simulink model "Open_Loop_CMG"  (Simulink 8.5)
settings: Solver=ode45  StartTime=0.0  StopTime=10.0  RelTol=1e-3
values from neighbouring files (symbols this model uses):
  Ave = [    [vehicle_flex34.m]    (also in vehicle_rigid.m)
  Bve = [    [vehicle_flex34.m]    (also in vehicle_rigid.m)
  Cve = [    [vehicle_flex34.m]    (also in vehicle_rigid.m)
  Dve = [    [vehicle_flex34.m]    (also in vehicle_rigid.m)
  J = [0.119416e9, -0.476e7,   -0.1216e7;     -0.476e7,     0.40408e8, -0.30121e6;     -0.1216e7,   -0.30121e6,  0.110166e9]    [start.m]    (also in start1.m; start2.m; start3.m)
  omg = 20*wo    (= 0.022)    [start.m]    (also in start1.m; start2.m; start3.m)
  zeb = 0.95    [start.m]    (also in start1.m; start2.m; start3.m)

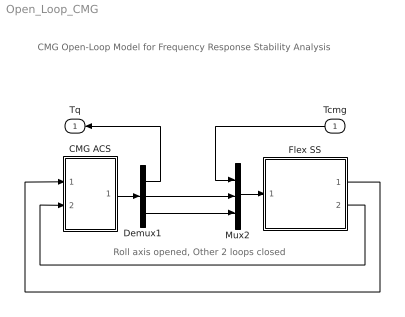
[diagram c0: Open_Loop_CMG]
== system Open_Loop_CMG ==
  note: CMG Open-Loop Model for Frequency Response Stability Analysis
  note: Roll axis opened, Other 2 loops closed
  Tcmg : Inport
  CMG ACS : Subsystem
  Demux1 : Demux  Outputs=3
  Flex SS : Subsystem
  Mux2 : Mux  Inputs=3
  Tq : Outport
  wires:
  Flex SS/2(att) -> CMG ACS/2(ater)
  Flex SS/1(wb) -> CMG ACS/1(wb)
  Mux2/1 -> Flex SS/1(Tcmg)
  CMG ACS/1(Tq) -> Demux1/1
  Demux1/2 -> Mux2/2
  Demux1/3 -> Mux2/3
  Demux1/1 -> Tq/1
  Tcmg/1 -> Mux2/1

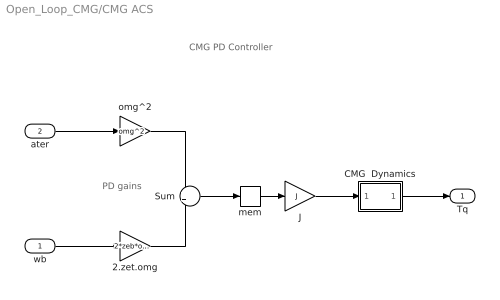
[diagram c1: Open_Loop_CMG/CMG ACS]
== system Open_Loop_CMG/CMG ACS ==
  note: CMG PD Controller
  note: PD gains
  wb : Inport
  ater : Inport  Port=2  PortDimensions=3
  2.zet.omg : Gain  Gain=2*zeb*omg
  CMG  Dynamics : Subsystem
  J : Gain  Gain=J  Multiplication=Matrix(K*u)
  Sum : Sum
  mem : Memory
  omg^2 : Gain  Gain=omg^2
  Tq : Outport
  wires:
  wb/1 -> 2.zet.omg/1
  Sum/1 -> mem/1
  2.zet.omg/1 -> Sum/2
  ater/1 -> omg^2/1
  omg^2/1 -> Sum/1
  J/1 -> CMG  Dynamics/1(I)
  mem/1 -> J/1
  CMG  Dynamics/1(O) -> Tq/1

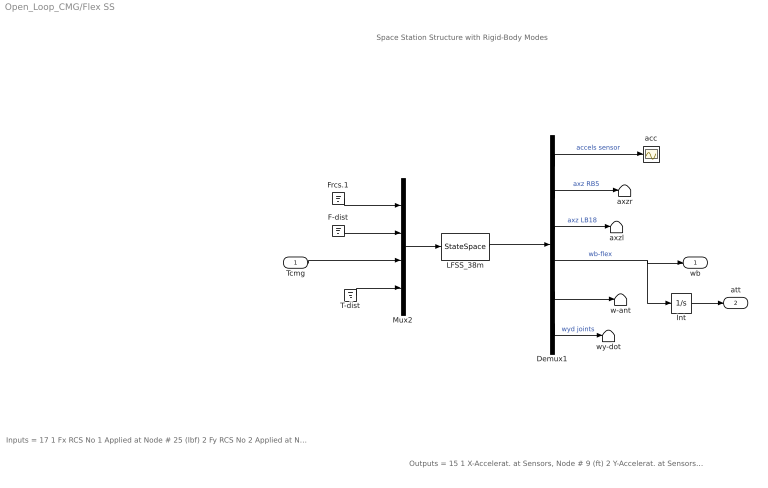
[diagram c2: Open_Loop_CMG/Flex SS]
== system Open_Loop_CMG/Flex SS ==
  note: Space Station Structure with Rigid-Body Modes
  note: Inputs = 17 1 Fx RCS No 1 Applied at Node # 25 (lbf) 2 Fy RCS No 2 Applied at Node # 25 (lbf) 3 Fx RCS No 3 Applied at Node # 26 (lbf) 4 Fy RCS No 4 Applied at Node # 26 (lbf) 5 Fx RCS No 5 Applied at Node # 27 (lbf) 6 Fy RCS No 6 Applied at Node # 27 (lbf) 7 Fx RCS No 7 Applied at Node # 28 (lbf) 8 Fy RCS No 8 Applied at Node # 28 (lbf) 9 Fx Disturb. No 9 at Node # 21 (lbf) 10 Fy Disturb. No 10 at Node # 21 (lbf) 11 Fz Disturb. No 11 at Node # 21 (lbf) 12 Torq-x No 1 CMG Applied at Node # 10 (ft-lb) 13 Torq-y No 2 CMG Applied at Node # 10 (ft-lb) 14 Torq-z No 3 CMG Applied at Node # 10 (ft-lb) 15 Torq-x No 4 Gimbal Dist. at Node # 1 (ft-lb) 16 Torq-y No 5 Gimbal Dist. at Node # 1 (ft-lb) 17 Torq-z No 6 Gimbal Dist. at Node # 1 (ft-lb)
  note: Outputs = 15 1 X-Accelerat. at Sensors, Node # 9 (ft) 2 Y-Accelerat. at Sensors, Node # 9 (ft) 3 Z-Accelerat. at Sensors, Node # 9 (ft) 4 X-Accelerat. at Right Boom End, Node # 5 (ft) 5 Z-Accelerat. at Right Boom End, Node # 5 (ft) 6 X-Accelerat. at Left Boom End, Node # 18 (ft) 7 Z-Accelerat. at Left Boom End, Node # 18 (ft) 8 X-Rot. Rate at Sensors, Node # 9 (radian) 9 Y-Rot. Rate at Sensors, Node # 9 (radian) 10 Z-Rot. Rate at Sensors, Node # 9 (radian) 11 X-Rot. Rate at Antena Bot-Left, Node # 24 (radian) 12 Y-Rot. Rate at Antena Bot-Left, Node # 24 (radian) 13 Z-Rot. Rate at Antena Bot-Left, Node # 24 (radian) 14 Y-Rot.Accel. at Right Joint, Node # 7 (radian) 15 Y-Rot.Accel. at Left Joint, Node # 16 (radian)
  Tcmg : Inport
  Demux1 : Demux  Outputs=[3, 2, 2, 3, 3, 2]
  F-dist : Ground
  Frcs.1 : Ground
  Int : Integrator
  LFSS_38m : StateSpace  A=Ave  B=Bve  C=Cve  D=Dve  X0=0
  Mux2 : Mux  Inputs=[8, 3, 3, 3]
  T-dist : Ground
  acc : Scope
  axzl : Terminator
  axzr : Terminator
  w-ant : Terminator
  wy-dot : Terminator
  wb : Outport
  att : Outport  Port=2
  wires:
  Int/1 -> att/1
  Mux2/1 -> LFSS_38m/1
  LFSS_38m/1 -> Demux1/1
  Demux1/1 -> acc/1  "accels sensor"
  Demux1/4 -> wb/1, Int/1  "wb-flex"
  Tcmg/1 -> Mux2/3
  Demux1/2 -> axzr/1  "axz RB5"
  Demux1/3 -> axzl/1  "axz LB18"
  F-dist/1 -> Mux2/2
  T-dist/1 -> Mux2/4
  Demux1/5 -> w-ant/1
  Demux1/6 -> wy-dot/1  "wyd joints"
  Frcs.1/1 -> Mux2/1

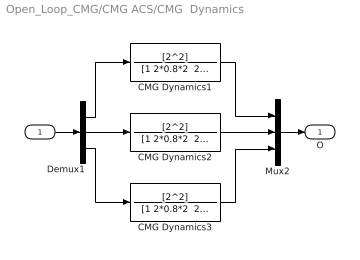
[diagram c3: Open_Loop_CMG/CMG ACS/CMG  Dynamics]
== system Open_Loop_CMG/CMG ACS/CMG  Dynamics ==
  I : Inport
  CMG Dynamics1 : TransferFcn  Numerator=[2^2]  Denominator="[1 2*0.8*2  2^2]"
  CMG Dynamics2 : TransferFcn  Numerator=[2^2]  Denominator="[1 2*0.8*2  2^2]"
  CMG Dynamics3 : TransferFcn  Numerator=[2^2]  Denominator="[1 2*0.8*2  2^2]"
  Demux1 : Demux  Outputs=3
  Mux2 : Mux  Inputs=3
  O : Outport
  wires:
  CMG Dynamics2/1 -> Mux2/2
  CMG Dynamics3/1 -> Mux2/3
  CMG Dynamics1/1 -> Mux2/1
  Demux1/2 -> CMG Dynamics2/1
  Demux1/1 -> CMG Dynamics1/1
  Demux1/3 -> CMG Dynamics3/1
  I/1 -> Demux1/1
  Mux2/1 -> O/1
